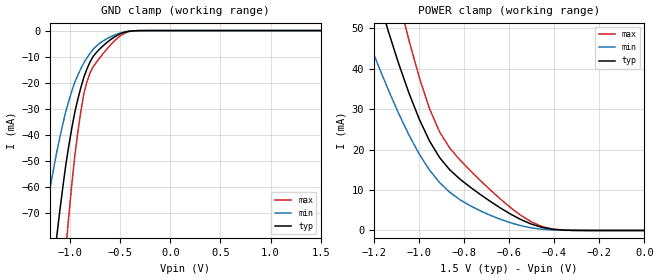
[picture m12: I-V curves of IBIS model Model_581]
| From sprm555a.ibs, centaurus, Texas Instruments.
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| Model based on original model for BCSHTLTCSCDDVPBFZ_SSGFV
|   Sub model DIFF_VREF_NOTERM_PUPD_OFF_10PER_1P5
[model]   Model_581
|[Description]  [1.5V-INPUT-PI-X, IND, 10%]
|   Weak pull up/down disabled,Industrial temperature range (-40C to
|   125C, 25C nominal),10% power supply tolerance
|[Input Load]   PI
|[Output Drive]
|Voltage   1.5V
|Mode   INPUT
Model_type   Input
Polarity   Non-Inverting
Vinl =  0.65
Vinh =  0.85
C_comp   1.865048p   1.676829p   1.989968p
[Model Spec]
Vinl   0.65   0.575   0.725
Vinh   0.85   0.775   0.925
[Temperature Range]   25   125   -40
[Voltage Range]   1.5   1.35   1.65
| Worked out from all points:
|   GND clamp passes 1 mA (typ) near -0.49 V on its own axis
|   POWER clamp passes 1 mA (typ) near -0.47 V on its own axis
[POWER_clamp]
-1.5V     126mA      88.79mA    168.8mA
-1.242V   69.83mA    49.45mA    94.45mA
-1.136V   49.22mA    34.73mA    67.74mA
-1.061V   36.46mA    25.42mA    50.44mA
-1V       27.61mA    18.95mA    38.01mA
-954.5mV  22.21mA    14.99mA    30.24mA
-909.1mV  18.03mA    11.85mA    24.36mA
-818.2mV  12.67mA    7.594mA    17.41mA
-590.9mV  3.954mA    1.85mA     5.519mA
-454.5mV  772.9uA    302.9uA    975.5uA
-363.6mV  110.4uA    48.27uA    110.4uA
0V        1.601nA    15.39nA    3.069nA
[GND_clamp]
-1.5V     -219.4mA   -131.6mA   -364.5mA
-1.288V   -134.6mA   -79.79mA   -225.8mA
-1.258V   -123.1mA   -72.83mA   -206.6mA
-1.136V   -79.49mA   -46.96mA   -132.6mA
-1.045V   -51.76mA   -31.17mA   -84.44mA
-1.015V   -44.3mA    -27.02mA   -71.26mA
-954.5mV  -31.3mA    -19.84mA   -47.97mA
-863.6mV  -17.79mA   -12.31mA   -24.03mA
-803mV    -12.1mA    -8.749mA   -16.28mA
-681.8mV  -6.163mA   -4.204mA   -9.294mA
-378.8mV  -129.8uA   -135.7uA   -184.8uA
1.5V      1.601nA    237.7nA    1.442nA
